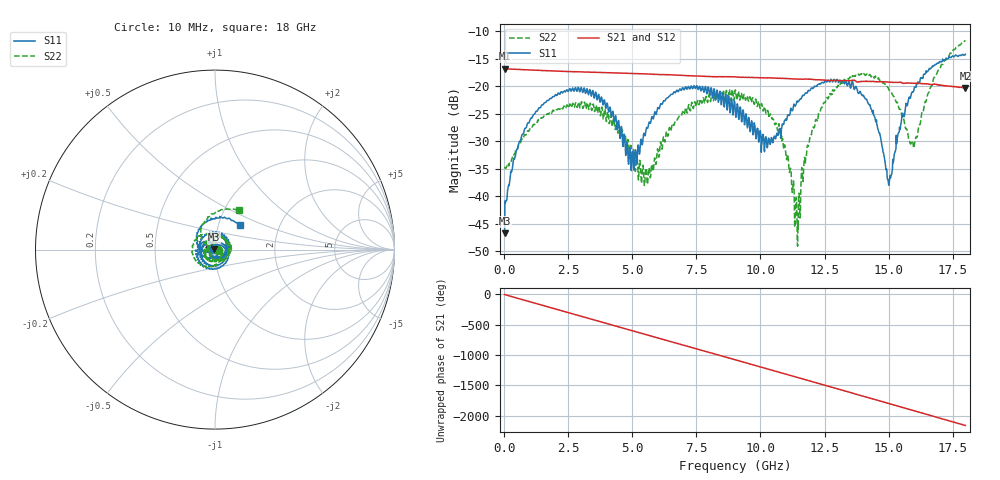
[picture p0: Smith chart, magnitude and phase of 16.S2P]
!Agilent Technologies,E5071C,MY46316741,A.11.02
!Date: Tue Sep 22 10:35:34 2020
!Data & Calibration Information:
!Freq	S11:SOLT4(ON)	S21:SOLT4(ON)	S12:SOLT4(ON)	S22:SOLT4(ON)
!PortZ  Port1:50+j0  Port2:50+j0
!Above PortZ is port z conversion or system Z0 setting when saving the data.
!When reading, reference impedance value at option line is always used.
# Hz S dB R 50
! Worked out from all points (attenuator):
!   1561 points, 10 MHz to 18 GHz, reference 50 ohm
!   highest |S21| = -16.84 dB at 10 MHz (marker M1); lowest = -20.3 dB at 18 GHz (marker M2)
!   lowest |S11| = -46.7 dB at 10 MHz (marker M3), VSWR 1.01, Z = 49.5 + j0.0653 ohm
!   |S11| at or under -10 dB: start of sweep to end of sweep
!   |S22| runs from -49.1 to -11.7 dB; largest |S21 - S12| = 0.0037
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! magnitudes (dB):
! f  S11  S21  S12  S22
! 10 MHz  -46.7  -16.8  -16.9  -34.9
! 402.1 MHz  -33.1  -16.9  -17.0  -32.4
! 967.2 MHz  -26.6  -17.1  -17.1  -28.1
! 3.02 GHz  -20.5  -17.4  -17.4  -22.9
! 4.069 GHz  -24.7  -17.6  -17.6  -25.7
! 5.003 GHz  -31.8  -17.7  -17.7  -33.6
! 5.522 GHz  -28.2  -17.8  -17.8  -34.9
! 6.007 GHz  -23.9  -17.9  -17.9  -31.9
! 7.264 GHz  -20.3  -18.1  -18.1  -24.5
! 9.005 GHz  -23.5  -18.3  -18.4  -20.9
! 10.1 GHz  -28.8  -18.5  -18.5  -24.5
! 10.67 GHz  -28.6  -18.5  -18.6  -28.0
! 11.12 GHz  -25.3  -18.6  -18.7  -35.1
! 11.4 GHz  -23.1  -18.7  -18.7  -40.6
! 12.01 GHz  -20.4  -18.8  -18.8  -28.0
! 12.89 GHz  -18.8  -19.0  -19.0  -20.8
! 14.08 GHz  -22.2  -19.1  -19.2  -17.9
! 14.48 GHz  -26.1  -19.2  -19.2  -18.2
! 15 GHz  -37.8  -19.3  -19.3  -20.5
! 15.95 GHz  -21.1  -19.5  -19.5  -30.3
! 16.82 GHz  -16.1  -19.6  -19.8  -18.3
! 18 GHz  -14.2  -20.3  -20.4  -11.7
